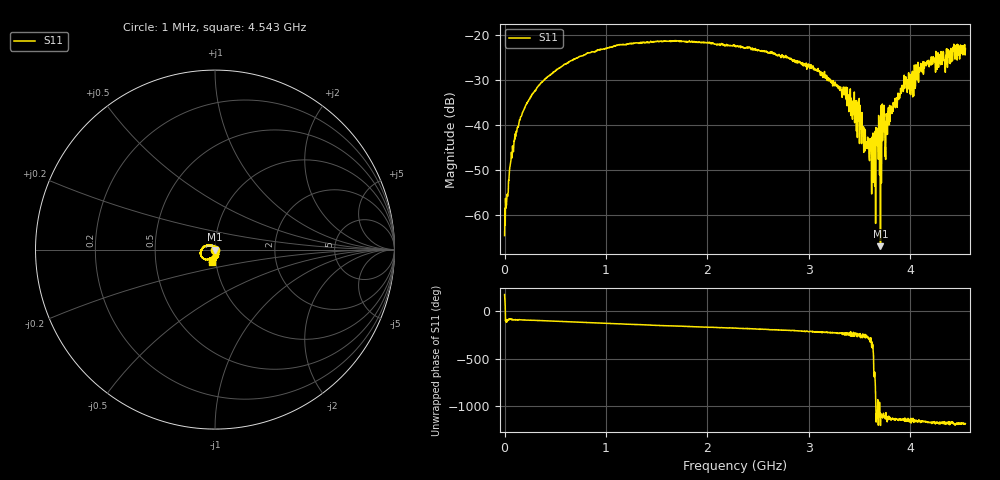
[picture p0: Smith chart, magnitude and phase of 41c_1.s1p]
# HZ S RI R 50
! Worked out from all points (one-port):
!   1515 points, 1 MHz to 4.543 GHz, reference 50 ohm
!   lowest |S11| = -66.9 dB at 3.706 GHz (marker M1), VSWR 1.00, Z = 50 - j0.0366 ohm
!   |S11| at or under -10 dB: start of sweep to end of sweep
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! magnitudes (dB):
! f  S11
! 1 MHz  -64.6
! 64 MHz  -47.8
! 115 MHz  -41.4
! 166 MHz  -38.1
! 340 MHz  -31.2
! 571 MHz  -27.0
! 1.138 GHz  -22.2
! 1.705 GHz  -21.4
! 2.272 GHz  -22.4
! 2.842 GHz  -25.9
! 3.154 GHz  -28.2
! 3.409 GHz  -32.0
! 3.502 GHz  -35.6
! 3.556 GHz  -41.1
! 3.637 GHz  -52.8
! 3.682 GHz  -42.4
! 3.685 GHz  -47.7
! 3.706 GHz  -66.9
! 3.73 GHz  -38.7
! 3.736 GHz  -36.3
! 3.742 GHz  -35.7
! 3.772 GHz  -42.0
! 3.799 GHz  -39.3
! 3.976 GHz  -30.0
! 4.015 GHz  -28.6
! 4.057 GHz  -26.7
! 4.156 GHz  -26.7
! 4.543 GHz  -23.1
